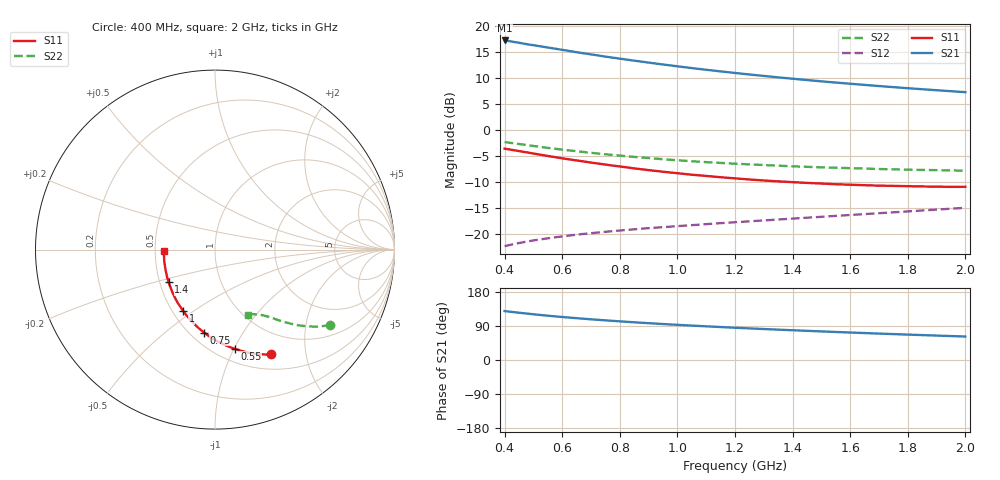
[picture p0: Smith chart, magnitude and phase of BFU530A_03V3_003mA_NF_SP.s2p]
! Filename:  P:\Prog\Test\Noise\ATS_data\Testdata_Net\06 Compressed Noise after Statistics\BFU530A_APG2013_33_A05_03p3V_003mA_NF_CM01_D.sf
! Date/Time: Tue 16/Apr/2013 15:10:54
! BFU530A_APG2013_33_A05_03p3V_1to25mA_NF_CM01_Bias3_R.sf
! Noise Parameter Data File
! BFU530A_APG2013_33_A05_03p3V_1to25mA_NF_CM01
! Date/time: Fri Apr 12 14:21:19 2013
! VAR V_out= 3.300000
! VAR I_out= 2.995000
! VAR V_in= 0.811200
! VAR I_in= 0.032005
! Device data file deembeded for feedlines and parallel
! Original file: \06 Compressed Noise after Statistics\BFU530A_APG2013_33_A05_03p3V_003mA_NF_CM01_R.sf
! Feed-files: PR017V01_150413_Feed1.s2p, PR017V01_150413_Feed2.s2p
! Parallel-file: PR017V01_150413_Par.s2p
# MHz S MA R 50
!  Freq-MHz  S11-mag  S11-arg  S21-mag  S21-arg  S12-mag  S12-arg  S22-mag  S22-arg
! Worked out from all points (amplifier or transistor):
!   37 points, 400 MHz to 2 GHz, reference 50 ohm
!   highest |S21| = 17.2 dB at 400 MHz (marker M1)
!   |S21| within 3 dB of that: start of sweep to 737.9 MHz
!   unconditionally stable (mu >= 1): 1.829 GHz to end of sweep
!   at 500 MHz: K = 0.44, MSG = 18.8 dB, |S12| = -21.2 dB
!   at 1.1 GHz: K = 0.81, MSG = 14.8 dB, |S12| = -18.1 dB
!   at 2 GHz: K = 1.01, MAG = 10.4 dB, |S12| = -14.9 dB
!   lowest NFmin = 0.52 dB at 420 MHz
!   S11 on the Smith chart (normalised r, x): 400 MHz: 0.69, -1.44; 550 MHz: 0.62, -1.01; 750 MHz: 0.58, -0.69; 1 GHz: 0.57, -0.45; 1.4 GHz: 0.56, -0.23; 2 GHz: 0.56, -0.01
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400  0.6634 -61.7  7.262 129.2  0.0767 59.5  0.7674 -33.1
420  0.6492 -64.2  7.118 127.3  0.07901 58.7  0.7538 -34.1
440  0.6355 -66.6  6.969 125.6  0.08118 57.9  0.7411 -35.0
480  0.6093 -71.1  6.668 122.3  0.08522 56.6  0.7159 -36.8
550  0.5639 -78.8  6.216 116.9  0.09123 54.6  0.6742 -39.4
600  0.5356 -83.8  5.9 113.5  0.0952 53.6  0.6488 -40.9
650  0.5111 -88.5  5.598 110.4  0.09901 52.8  0.6267 -42.3
700  0.4874 -93.2  5.338 107.4  0.1022 52.1  0.605 -43.6
750  0.4662 -97.5  5.08 104.6  0.1054 51.6  0.5857 -44.6
800  0.4471 -101.7  4.856 102.0  0.1085 51.3  0.5685 -45.6
850  0.4288 -105.9  4.644 99.5  0.1114 51.0  0.5523 -46.6
900  0.4124 -110.0  4.449 97.1  0.1143 50.8  0.5389 -47.4
950  0.3979 -113.8  4.268 94.9  0.1168 50.8  0.5249 -48.3
1000  0.3851 -117.5  4.1 92.8  0.1195 50.8  0.5133 -49.0
1100  0.3627 -124.8  3.798 88.9  0.1248 51.0  0.4922 -50.4
1200  0.3438 -131.7  3.538 85.2  0.1302 51.3  0.4754 -51.7
1300  0.328 -138.3  3.313 81.7  0.1356 51.7  0.4615 -53.1
1400  0.3162 -144.8  3.115 78.5  0.1411 52.2  0.449 -54.4
1500  0.3065 -151.1  2.94 75.4  0.1468 52.7  0.4387 -55.7
1650  0.2954 -159.8  2.717 71.1  0.1559 53.5  0.4268 -57.8
1750  0.2909 -165.4  2.585 68.3  0.1622 54.1  0.4195 -59.0
2000  0.2851 -178.4  2.314 61.9  0.1792 55.2  0.4078 -62.8
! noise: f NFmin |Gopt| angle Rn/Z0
400  0.5634  0.3525  19.55  0.1552
460  0.5674  0.3246  29.28  0.1417
600  0.6449  0.3265  30.31  0.1549
800  0.6417  0.3066  52.28  0.125
1000  0.6813  0.3008  67.29  0.1155
1200  0.7186  0.291  82.17  0.1112
1400  0.7658  0.2823  97.78  0.0957
1600  0.7952  0.2631  117.1  0.0869
1800  0.7223  0.3047  137.4  0.0669
2000  0.754  0.3134  147  0.0625
